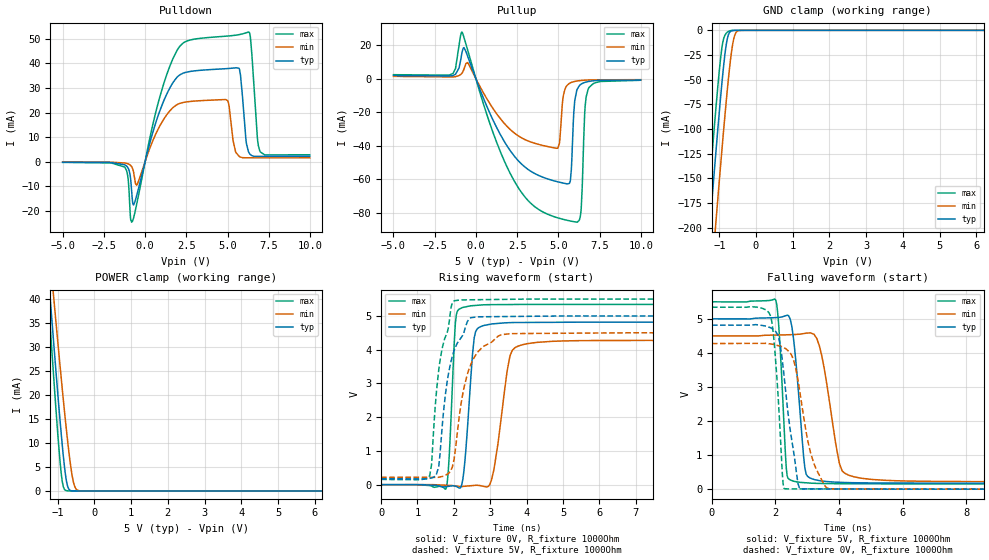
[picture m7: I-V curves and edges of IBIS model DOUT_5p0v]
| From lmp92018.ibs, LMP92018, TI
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|   Model
[Model]   DOUT_5p0v
Model_type   3-state
Polarity   Non-Inverting
Vmeas = 2.5
Vref = 0
Cref = 1pF
Rref = 1000000
|   typ   min   max
C_comp   0.5310pF   0.5030pF   0.6389pF
[Voltage Range]   5   4.5   5.5
[Temperature Range]   27   125   -40
[Pullup Reference]   5   4.5   5.5
[Pulldown Reference]   0   0   0
[Power Clamp Reference]   5   4.5   5.5
[GND Clamp Reference]   0   0   0
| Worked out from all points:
|   slope of the pulldown table from 0 to 0.75 V, typ, clamps not added: 41.7 ohm
|   slope of the pullup table from 0 to 0.75 V, typ, clamps not added: 40.7 ohm
|   GND clamp passes 1 mA (typ) near -0.69 V on its own axis
|   POWER clamp passes 1 mA (typ) near -0.73 V on its own axis
|   falling waveform, V_fixture 5V, R_fixture 1000Ohm: 20-80 % time 257ps typ, 434ps min, 174ps max; typ from 5 V to 0.176 V
|   rising waveform, V_fixture 0V, R_fixture 1000Ohm: 20-80 % time 187ps typ, 313ps min, 131ps max; typ from 0 V to 4.82 V
|   rising waveform, V_fixture 5V, R_fixture 1000Ohm: 20-80 % time 391ps typ, 452ps min, 364ps max; typ from 0.176 V to 5 V
|   falling waveform, V_fixture 0V, R_fixture 1000Ohm: 20-80 % time 387ps typ, 511ps min, 219ps max; typ from 4.82 V to 0 V
[Pulldown]
|   Voltage   I(typ)   I(min)   I(max)
-5V       -189.4uA   -99uA      -265.2uA
-1.235V   -1.241mA   -519uA     -2.178mA
-815mV    -11.91mA   -2.005mA   -24.6mA
-485mV    -13.1mA    -9.296mA   -16.45mA
865mV     20.19mA    14.24mA    25.71mA
2.335V    36.11mA    24.14mA    48.44mA
5.005V    37.92mA    24.89mA    51.15mA
5.695V    38.06mA    2.241mA    51.72mA
6.265V    4.148mA    1.6mA      52.75mA
6.385V    2.902mA    1.6mA      50.64mA
6.955V    2.176mA    1.601mA    4.392mA
9.985V    2.198mA    1.608mA    2.821mA
[GND Clamp]
|   Voltage   I(typ)   I(min)   I(max)
-5V       -2.033A    -2.097A    -1.993A
-1.355V   -245.8mA   -317.6mA   -200.4mA
-1.295V   -217.4mA   -289.3mA   -172.1mA
-1.235V   -189.3mA   -261.1mA   -144mA
-1.085V   -120.6mA   -191.7mA   -76.36mA
-965mV    -68.57mA   -137.6mA   -28.86mA
-905mV    -44.74mA   -111.4mA   -12.44mA
-815mV    -15.62mA   -73.86mA   -3.197mA
-725mV    -2.425mA   -40.01mA   -665.1uA
-605mV    -132.3uA   -8.467mA   -27.41uA
-425mV    -885.7nA   -94.72uA   0A
9.985V    0A         0A         0A
[Pullup]
|   Voltage   I(typ)   I(min)   I(max)
-5V       1.954mA    1.416mA    2.417mA
-1.385V   1.884mA    1.081mA    3.155mA
-845mV    15.39mA    3.351mA    27.81mA
1.915V    -40.43mA   -28.66mA   -53.13mA
4.435V    -59.97mA   -40.59mA   -81.1mA
4.975V    -61.45mA   -41.26mA   -82.94mA
5.695V    -61.85mA   -2.623mA   -84.72mA
6.115V    -6.948mA   -1.362mA   -85.5mA
6.385V    -3.196mA   -1.026mA   -77.38mA
6.595V    -2.211mA   -857.4uA   -20.93mA
6.805V    -1.678mA   -734.2uA   -6.277mA
9.985V    -784.3uA   -554uA     -905.6uA
[POWER Clamp]
|   Voltage   I(typ)   I(min)   I(max)
-5V       421.2mA    372.4mA    477.1mA
-1.265V   46.43mA    53.79mA    41.59mA
-1.205V   40.46mA    48.67mA    34.71mA
-1.115V   31.63mA    41.05mA    24.58mA
-905mV    12.16mA    23.77mA    3.859mA
-845mV    7.297mA    19.05mA    864uA
-785mV    3.293mA    14.51mA    130uA
-725mV    879uA      10.22mA    26.23uA
-605mV    19.33uA    3.196mA    0A
-515mV    0A         602.4uA    0A
-425mV    0A         61.71uA    0A
9.985V    0A         0A         0A
[Ramp]
R_load = 1000
|   typ   min   max
dV/dt_r   2.88949/1.87052e-10   2.56466/3.12893e-10   3.20541/1.31463e-10
dV/dt_f   2.89413/2.571e-10   2.56851/4.33665e-10   3.2068/1.74417e-10
[Falling Waveform]
V_fixture = 5V
V_fixture_min = 4.5V
V_fixture_max = 5.5V
R_fixture = 1000Ohm
C_fixture = 0F
|   Time   V(typ)   V(min)   V(max)
0s        5V         4.5V       5.5V
2.008ns   5.037V     4.524V     5.552V
2.411ns   5.096V     4.534V     308.6mV
2.596ns   4.197V     4.54V      229mV
2.925ns   620.8mV    4.574V     189.6mV
3.114ns   318mV      4.584V     176.8mV
3.464ns   239.8mV    3.891V     166.6mV
4.099ns   198.3mV    535mV      158.6mV
5.401ns   180.7mV    262.5mV    156.1mV
100ns     176.5mV    219.1mV    155.3mV
[Rising Waveform]
V_fixture = 0V
V_fixture_min = 0V
V_fixture_max = 0V
R_fixture = 1000Ohm
C_fixture = 0F
|   Time   V(typ)   V(min)   V(max)
0s        -7.616uV   3.327uV    18.15uV
1.787ns   -57.87mV   -16.92mV   -109.8mV
2.041ns   -46.29mV   -37.66mV   4.787V
2.184ns   -87.26mV   -57.95mV   5.223V
2.558ns   4.348V     -22.19mV   5.308V
2.775ns   4.699V     -39.68mV   5.327V
3.101ns   4.769V     449.4mV    5.335V
3.603ns   4.804V     3.977V     5.339V
4.701ns   4.811V     4.248V     5.342V
100ns     4.816V     4.274V     5.342V
[Rising Waveform]
V_fixture = 5V
V_fixture_min = 4.5V
V_fixture_max = 5.5V
R_fixture = 1000Ohm
C_fixture = 0F
|   Time   V(typ)   V(min)   V(max)
0s        176.5mV    219.1mV    155.3mV
1.336ns   187.4mV    217.1mV    273.7mV
1.517ns   294.4mV    216.9mV    2.692V
1.641ns   1.207V     234.1mV    3.823V
1.783ns   2.804V     289.6mV    4.423V
1.955ns   3.796V     511.4mV    5.371V
2.183ns   4.332V     2.294V     5.474V
2.628ns   4.971V     3.897V     5.481V
3.603ns   4.984V     4.476V     5.494V
100ns     5V         4.5V       5.5V
[Falling Waveform]
|Gnd
V_fixture = 0V
V_fixture_min = 0V
V_fixture_max = 0V
R_fixture = 1000Ohm
C_fixture = 0F
|   Time   V(typ)   V(min)   V(max)
0s        4.816V     4.274V     5.342V
1.835ns   4.743V     4.265V     5.105V
2.008ns   4.625V     4.234V     3.74V
2.24ns    3.584V     4.164V     156.8mV
2.341ns   2.703V     4.111V     10.08mV
2.559ns   1.169V     3.819V     8.425mV
2.753ns   42.49mV    2.944V     7.91mV
3.213ns   7.45mV     743.2mV    6.688mV
3.735ns   6.122mV    10.6mV     5.3mV
100ns     -7.618uV   3.309uV    -18.17uV
